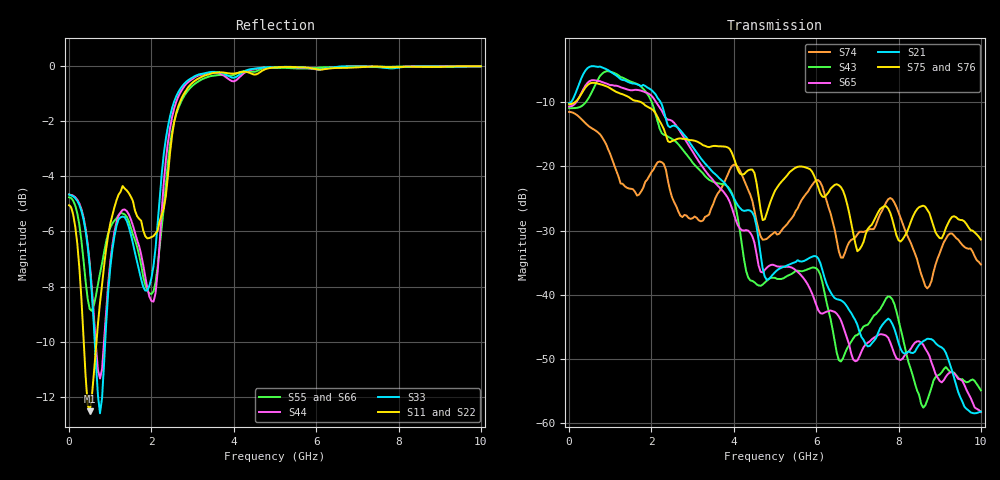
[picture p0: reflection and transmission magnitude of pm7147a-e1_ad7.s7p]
# GHz S DB R 50
! S-Parameters data
! Freq  dbS11  angS11  dbS12  angS12  dbS13  angS13  dbS14  angS14
!  dbS15  angS15  dbS16  angS16  dbS17  angS17  dbS21  angS21
!  dbS22  angS22  dbS23  angS23  dbS24  angS24  dbS25  angS25
!  dbS26  angS26  dbS27  angS27  dbS31  angS31  dbS32  angS32
!  dbS33  angS33  dbS34  angS34  dbS35  angS35  dbS36  angS36
!  dbS37  angS37  dbS41  angS41  dbS42  angS42  dbS43  angS43
!  dbS44  angS44  dbS45  angS45  dbS46  angS46  dbS47  angS47
!  dbS51  angS51  dbS52  angS52  dbS53  angS53  dbS54  angS54
!  dbS55  angS55  dbS56  angS56  dbS57  angS57  dbS61  angS61
!  dbS62  angS62  dbS63  angS63  dbS64  angS64  dbS65  angS65
!  dbS66  angS66  dbS67  angS67  dbS71  angS71  dbS72  angS72
!  dbS73  angS73  dbS74  angS74  dbS75  angS75  dbS76  angS76
!  dbS77  angS77
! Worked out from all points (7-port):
!   279 points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, 1 Hz to 10 GHz, reference 50 ohm
!   strongest paths, dB at 1 Hz, 7.943 MHz, 3.05 GHz, 6.55 GHz, 10 GHz:
!     S75: -10.3, -10.3, -16.0, -22.9, -31.4
!     S76: -10.3, -10.3, -16.1, -23.2, -31.7
!     S21: -10.2, -10.2, -17.4, -40.8, -58.2
!     S65: -10.7, -10.7, -18.3, -43.4, -58.3
!     S43: -11.0, -11.0, -19.8, -50.2, -54.9
!     S74: -11.5, -11.5, -27.8, -33.2, -35.3
!   lowest |S11| = -12.5 dB at 500 MHz (marker M1), VSWR 1.62, Z = 30.9 - j0.729 ohm
!   |S11| at or under -10 dB: 356 MHz to 664.6 MHz (308.6 MHz wide, 60.5 % of centre)
